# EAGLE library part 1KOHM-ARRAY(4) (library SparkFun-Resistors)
4 x 1kΩ resistor array A resistor is a passive two-terminal electrical component that implements electrical resistance as a circuit element. Resistors act to reduce current flow, and, at the same time, act to lower voltage levels within circuits. - Wikipedia An array is a collection of discrete resistors in a single package.
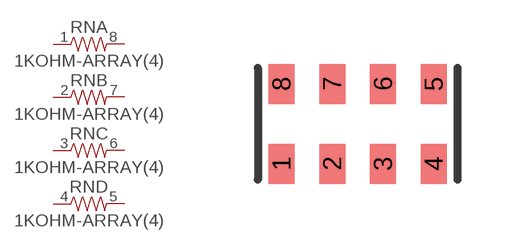
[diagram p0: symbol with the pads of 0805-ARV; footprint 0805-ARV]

Designator prefix RN; gates B=RESISTOR-PADS C=RESISTOR-PADS D=RESISTOR-PADS A=RESISTOR-PADS

## 1KOHM-ARRAY(4)-0805_ARV-1/10W-5% (PROD_ID: RES-13020; VALUE: 1k)  [0805-ARV]
1  A:1  pas
2  B:1  pas
3  C:1  pas
4  D:1  pas
5  D:2  pas
6  C:2  pas
7  B:2  pas
8  A:2  pas

## Footprint 0805-ARV (pad centres in mm)
4X2012(0805) resistor array
smd 0.65 x 1: 1 -1.905,-1; 2 -0.635,-1; 3 0.635,-1; 4 1.905,-1; 5 1.905,1; 6 0.635,1; 7 -0.635,1; 8 -1.905,1

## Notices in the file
Licensing: Creative Commons ShareAlike 4.0 International - https://creativecommons.org/licenses/by-sa/4.0
